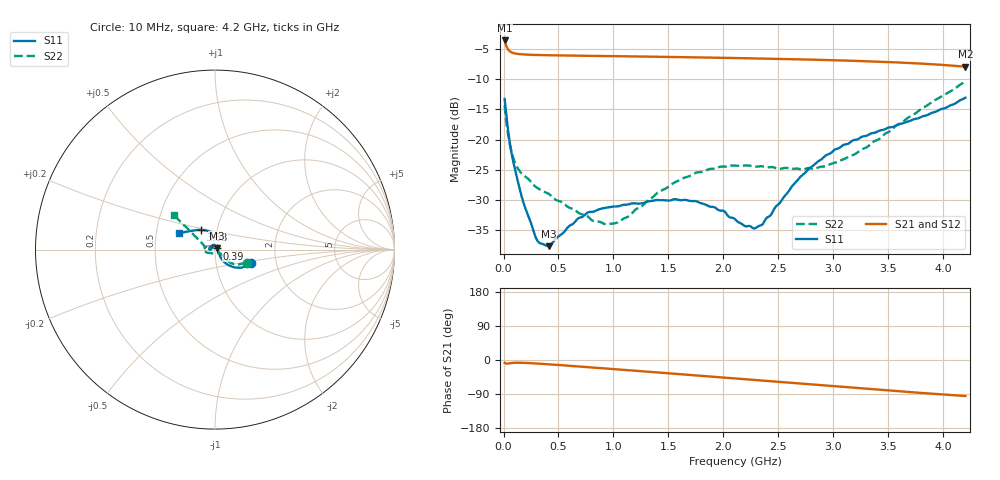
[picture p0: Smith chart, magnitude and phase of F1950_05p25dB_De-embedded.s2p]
! Integrated Device Technology
! Corporate Headquarters
! 6024 Silver Creek Valley Road
! San Jose, CA 95138  USA
! Phone:  1-408-284-8200
! Toll Free:  1-800-223-1366
! Webpage:  http://www.idt.com/
! Timing and RF Division
! 515 Groton Road, Suite 102
! Westford, MA 01886-6024
! Device:  F1950
! Description: 7-bit 0.25 dB Digital Step Attenuator
! Frequency:  150.0 -  4000.00 MHz
! Package:  4x4 mm Thin QFN Plastic Package: 24 pin
! Ports:  2 RF, 12 DC
!  Pin  1  = D0
!  Pin  2  = VDD
!  Pin  3  = Vmode
!  Pin  4  = GND
!  Pin  5  = RF1  =  Port 1
!  Pin  6  = GND
!  Pin  7  = GND
!  Pin  8  = GND
!  Pin  9  = GND
!  Pin 10  = GND
!  Pin 11  = GND
!  Pin 12  = GND
!  Pin 13  = GND
!  Pin 14  = RF2  =  Port 2
!  Pin 15  = GND
!  Pin 16  = LE
!  Pin 17  = CLK
!  Pin 18  = DATE
!  Pin 19  = D6
!  Pin 20  = D5
!  Pin 21  = D4
!  Pin 22  = D3
!  Pin 23  = D2
!  Pin 24  = D1
! State:  21
! Atten State:  5.25 dB
! Voltage:  +5.00 Volts
! Current:  Not Measured mA
! Data:  The device was measured on a the F195X evaluation board which has
!  individual transmission lines to the RF pins.  Data was collected
!  using a calibrated network analyzer.  The evaluation board was
!  de-embedded using a TRL calibration technique.
!  The reference plane is the edge of the package pin.
! Misc:  Board 2019
!  Action Tracker AT0250
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# GHz S dB R 50
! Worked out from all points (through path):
!   420 points, 10 MHz to 4.2 GHz, reference 50 ohm
!   highest |S21| = -3.66 dB at 10 MHz (marker M1); lowest = -8.0 dB at 4.2 GHz (marker M2)
!   group delay of S21, straight-line fit = 61.4 ps
!   lowest |S11| = -37.6 dB at 410 MHz (marker M3), VSWR 1.03, Z = 51.1 + j0.784 ohm
!   |S11| at or under -10 dB: start of sweep to end of sweep
!   |S22| runs from -34.0 to -10.4 dB; largest |S21 - S12| = 0.0013
!   S11 on the Smith chart (normalised r, x): 10 MHz: 1.48, -0.24; 390 MHz: 1.02, +0.01; 3.63 GHz: 0.83, +0.19; 4.2 GHz: 0.66, +0.13
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0.01  -13.31 -21.0  -3.66 -7.3  -3.65 -7.3  -14.37 -23.0
0.05  -19.63 -50.9  -5.32 -8.8  -5.32 -8.8  -20.12 -41.4
0.08  -22.92 -54.6  -5.68 -7.7  -5.67 -7.7  -22.51 -39.8
0.12  -26.08 -53.6  -5.85 -7.2  -5.85 -7.2  -24.45 -36.3
0.17  -29.69 -44.5  -5.95 -7.4  -5.95 -7.4  -25.72 -36.7
0.3  -36.42 -8.9  -6.05 -9.2  -6.05 -9.3  -27.90 -35.5
0.39  -37.52 27.7  -6.09 -10.9  -6.09 -11.0  -28.78 -36.5
0.41  -37.59 35.6  -6.09 -11.3  -6.10 -11.4  -28.95 -36.4
0.71  -32.81 99.4  -6.17 -17.6  -6.17 -17.7  -32.31 -52.6
0.92  -31.30 119.1  -6.23 -22.2  -6.23 -22.3  -33.94 -79.4
1.02  -31.05 127.2  -6.25 -24.4  -6.25 -24.5  -33.76 -98.6
1.41  -29.98 161.6  -6.35 -33.1  -6.35 -33.1  -28.65 -147.5
1.75  -30.16 -180.0  -6.44 -40.6  -6.44 -40.7  -25.48 -164.6
2.11  -33.22 171.7  -6.55 -48.7  -6.56 -48.8  -24.32 -175.9
2.27  -34.63 144.0  -6.61 -52.3  -6.61 -52.4  -24.43 -179.6
2.34  -34.18 130.3  -6.64 -53.9  -6.64 -54.0  -24.40 178.5
2.64  -27.38 95.2  -6.74 -60.7  -6.74 -60.8  -24.81 171.1
2.81  -24.38 93.8  -6.82 -64.6  -6.82 -64.7  -24.83 166.2
3.19  -20.07 104.7  -7.02 -73.3  -7.01 -73.4  -22.47 155.8
3.51  -18.00 120.0  -7.22 -80.5  -7.22 -80.7  -18.67 147.8
3.63  -17.32 126.2  -7.32 -83.2  -7.31 -83.4  -17.11 145.7
4.2  -13.10 155.0  -8.00 -94.9  -7.99 -95.1  -10.45 139.9
